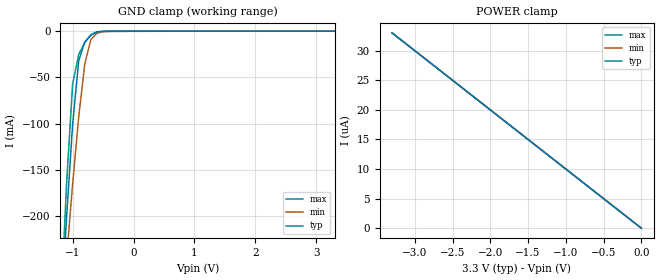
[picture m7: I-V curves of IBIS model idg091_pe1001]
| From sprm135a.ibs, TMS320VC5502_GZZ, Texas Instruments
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[Model]   idg091_pe1001
Model_type   Input
Polarity   Non-Inverting
| signals   A, Y
Vinl = 0.8V
Vinh = 2.0V
|   typ   min   max
C_comp   1.5639p   1.4731p   1.7754p
|   typ   min   max
[Temperature Range]   25   -40   125
|   typ   min   max
[Voltage Range]   3.30V   3.00V   3.60V
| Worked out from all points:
|   GND clamp passes 1 mA (typ) near -0.60 V on its own axis
[GND_clamp]
|   Voltage   I(typ)   I(min)   I(max)
-3.3V     -2.948A    -2.226A    -3.826A
-1.2V     -315mA     -329.1mA   -310.8mA
-1.1V     -202.2mA   -245.6mA   -165.7mA
-1V       -100.7mA   -165.6mA   -57.2mA
-900mV    -31.78mA   -92.55mA   -25.1mA
-800mV    -11.59mA   -35.39mA   -12.2mA
-700mV    -4.301mA   -8.684mA   -3.697mA
-600mV    -913.1uA   -2.172mA   -535.7uA
-500mV    -158.7uA   -440.6uA   -129.9uA
-400mV    -77.17uA   -101uA     -95.66uA
3.3V      100.3uA    54.94uA    173.6uA
[POWER_clamp]
|   Voltage   I(typ)   I(min)   I(max)
-3.3V     33uA       33uA       33uA
-3.2V     32uA       32.01uA    32uA
-100mV    1uA        1.003uA    1uA
0V        1pA        1pA        1pA
